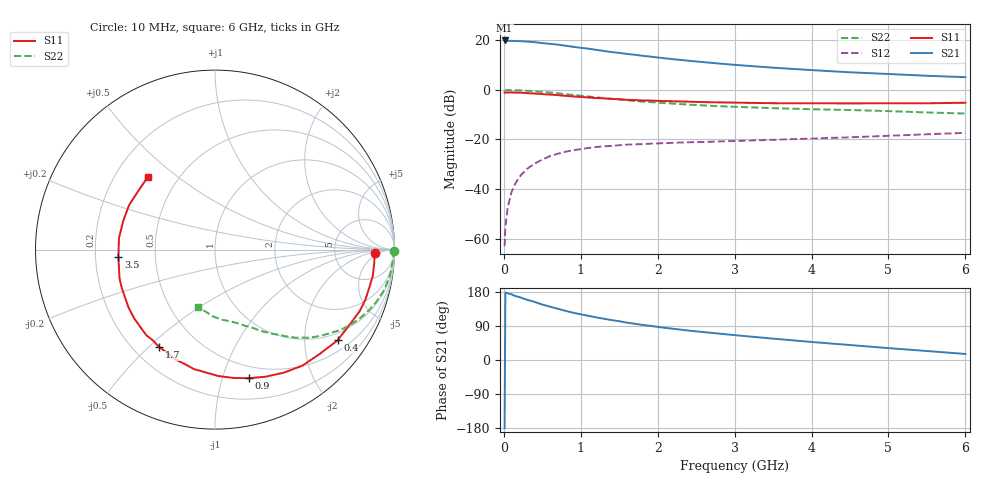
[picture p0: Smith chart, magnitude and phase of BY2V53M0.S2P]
! SIEMENS Small Signal Semiconductors
! BFY420
! Si NPN RF SIEGET Grounded Emitter Transistor in MICRO-X
! VCE = 2.5 V  IC = 3 mA
! Common Emitter S-Parameters:  October  1996
# GHz  S  MA  R  50
!  f  S11  S21  S12  S22
! GHz  MAG  ANG  MAG  ANG  MAG  ANG  MAG  ANG
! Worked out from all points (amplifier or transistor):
!   36 points, 10 MHz to 6 GHz, reference 50 ohm
!   highest |S21| = 20.0 dB at 10 MHz (marker M1)
!   |S21| within 3 dB of that: start of sweep to 1.01 GHz
!   unconditionally stable (mu >= 1): 3.635 GHz to end of sweep
!   at 250 MHz: K = 0.07, MSG = 26.6 dB, |S12| = -33.5 dB
!   at 1.4 GHz: K = 0.38, MSG = 19.0 dB, |S12| = -22.6 dB
!   at 6 GHz: K = 1.19, MAG = 8.6 dB, |S12| = -17.3 dB
!   S11 on the Smith chart (normalised r, x): 10 MHz: 17, -3; 400 MHz: 0.78, -2.84; 900 MHz: 0.39, -1.23; 1.7 GHz: 0.30, -0.54; 3.5 GHz: 0.30, -0.03; 6 GHz: 0.34, +0.40
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0.01  0.8896 -1.1  10 -179.8  0.0007 95.2  0.9954 -0.4
0.02  0.889 -2.2  9.998 178.1  0.0017 91.4  0.988 -0.9
0.05  0.8903 -4.6  9.826 175.9  0.0042 87.4  0.9942 -2.3
0.1  0.8913 -9.4  9.816 173.3  0.0087 85.0  0.9899 -4.7
0.15  0.8852 -13.9  9.735 168.7  0.0129 79.3  0.987 -7.2
0.2  0.8832 -18.5  9.702 166.2  0.0174 81.0  0.9826 -9.3
0.3  0.8624 -27.6  9.505 159.0  0.0254 75.0  0.9662 -14.0
0.4  0.8496 -36.5  9.241 153.3  0.0326 70.0  0.9423 -18.4
0.5  0.8238 -44.8  8.851 146.2  0.0393 65.8  0.916 -22.4
0.6  0.8093 -53.0  8.561 140.8  0.0463 61.6  0.8869 -26.2
0.7  0.7861 -60.6  8.23 135.2  0.0514 57.9  0.8578 -29.7
0.9  0.7412 -75.1  7.452 124.8  0.0609 50.7  0.7941 -35.8
1.1  0.7048 -88.5  6.819 116.5  0.0674 45.6  0.7382 -41.2
1.2  0.6864 -94.2  6.466 112.4  0.0704 43.4  0.7121 -43.6
1.4  0.6589 -105.0  5.82 105.4  0.0741 39.3  0.6661 -47.5
1.7  0.6258 -119.8  5.14 95.7  0.0796 34.8  0.599 -52.6
2.2  0.5912 -139.5  4.182 82.4  0.0857 29.6  0.5305 -59.5
2.8  0.5614 -157.7  3.418 69.6  0.0913 26.5  0.4694 -66.2
3.5  0.5398 -175.6  2.818 56.4  0.0986 24.5  0.4289 -73.0
4.5  0.5358 162.7  2.276 39.5  0.1107 22.1  0.3936 -83.9
5.5  0.5383 142.2  1.935 23.7  0.1273 19.1  0.3517 -97.9
6  0.5518 132.7  1.814 15.9  0.136 17.0  0.3339 -106.1
